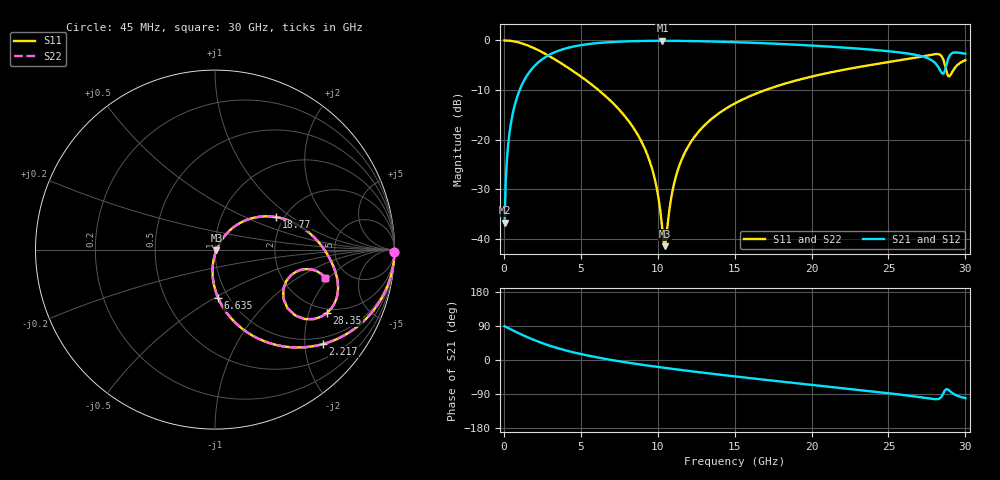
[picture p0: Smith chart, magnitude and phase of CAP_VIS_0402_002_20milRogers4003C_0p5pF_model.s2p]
! S-parameter model data by Modelithics Inc.  support@modelithics.com  813-866-6335  Tampa FL USA
! S-Parameter data specifications:
! Substrate: 20-mil Rogers 4003C, substrate thickness, H=0.508mm, Dielectric constant, Er=3.75
! PCB Mounting Pad Footprint: Pad width, PadW=0.50mm , Pad length, PadL=0.50mm , Pad gap, PadG (edge-to-edge)=0.40mm , Reference planes=1.4mm apart
! Created Wed Nov 18 12:41:05 2015
# hz S ma R 50
! 2 Port Network Data from SP1.SP block
! freq  magS11  angS11  magS21  angS21  magS12  angS12  magS22  angS22
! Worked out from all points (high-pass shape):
!   401 points, 45 MHz to 30 GHz, reference 50 ohm
!   highest |S21| = -0.08 dB at 10.3 GHz (marker M1); lowest = -36.8 dB at 45 MHz (marker M2)
!   |S21| within 3 dB of the highest: 2.848 GHz to 27.03 GHz (24.18 GHz wide, 162 % of centre); 28.98 GHz to end of sweep
!   lowest |S11| = -41.5 dB at 10.45 GHz (marker M3), VSWR 1.02, Z = 50.8 - j0.308 ohm
!   |S11| at or under -10 dB: 6.145 GHz to 17 GHz (10.86 GHz wide, 93.8 % of centre)
!   |S22| runs from -41.5 to 0.0 dB; largest |S21 - S12| = 0
!   S11 on the Smith chart (normalised r, x): 45 MHz: open; 2.217 GHz: 0.83, -2.42; 6.635 GHz: 0.89, -0.52; 18.77 GHz: 1.82, +0.77; 28.35 GHz: 1.83, -2.65; 30 GHz: 3.45, -1.79
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4.5e7  0.9999 -0.9  0.01453 89.1  0.01453 89.1  0.9999 -0.9
3.4455e8  0.9938 -7.0  0.1107 82.9  0.1107 82.9  0.9938 -7.0
6.441e8  0.9788 -13.1  0.2043 76.9  0.2043 76.9  0.9788 -13.1
1.2432e9  0.9259 -24.6  0.3767 65.3  0.3767 65.3  0.9259 -24.6
2.216738e9  0.7998 -41.1  0.598 48.7  0.598 48.7  0.7998 -41.1
5.062462e9  0.4262 -74.2  0.8994 15.1  0.8994 15.1  0.4262 -74.2
6.6351e9  0.2718 -86.1  0.9559 2.6  0.9559 2.6  0.2718 -86.1
8.956612e9  0.09439 -97.8  0.9877 -12.4  0.9877 -12.4  0.09439 -97.8
9.6306e9  0.05085 -97.3  0.9905 -16.3  0.9905 -16.3  0.05085 -97.3
1.007992e10  0.02388 -88.7  0.9912 -18.8  0.9912 -18.8  0.02388 -88.7
1.030459e10  0.0122 -67.0  0.9913 -20.0  0.9913 -20.0  0.0122 -67.0
1.045436e10  0.008402 -21.2  0.9913 -20.8  0.9913 -20.8  0.008402 -21.2
1.112835e10  0.03956 52.9  0.9902 -24.4  0.9902 -24.4  0.03956 52.9
1.180234e10  0.07592 55.3  0.9877 -27.8  0.9877 -27.8  0.07592 55.3
1.50225e10  0.2319 44.1  0.9618 -43.4  0.9618 -43.4  0.2319 44.1
1.876688e10  0.3858 28.0  0.9098 -60.2  0.9098 -60.2  0.3858 28.0
2.003996e10  0.4333 22.5  0.8878 -65.8  0.8878 -65.8  0.4333 22.5
2.505742e10  0.6065 0.3  0.777 -88.0  0.777 -88.0  0.6065 0.3
2.835248e10  0.7167 -29.5  0.5013 -100.6  0.5013 -100.6  0.7167 -29.5
2.887669e10  0.4392 -29.9  0.6511 -78.1  0.6511 -78.1  0.4392 -29.9
2.925112e10  0.5116 -12.3  0.7546 -89.8  0.7546 -89.8  0.5116 -12.3
3e10  0.6326 -14.2  0.7348 -100.7  0.7348 -100.7  0.6326 -14.2
